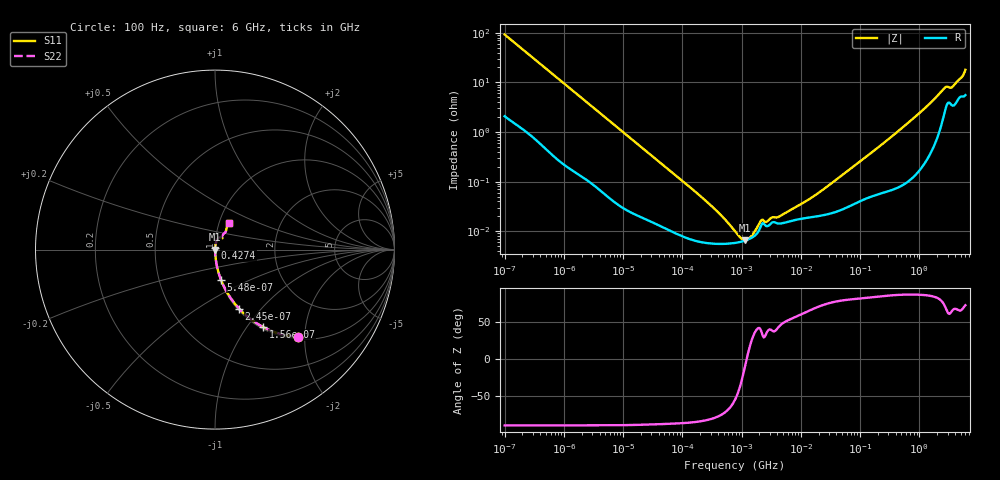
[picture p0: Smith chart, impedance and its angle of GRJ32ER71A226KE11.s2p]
!Murata Part Number: GRJ32ER71A226KE11
!These Parameters are Measured in Series Mode Connection
!Data Generated on Jun 19, 2026
!  o--ll--o
!Port1  Port2
!  o------o
!Operation Temp=25[degC], DC Bias Voltage=0[V]
!Freq. Start=100[Hz] Stop=6[GHz] 401[Steps]
# Hz S RI R 50
!Freq.(Hz) S11(Real) S11(Imag) S21(Real) S21(Imag) S12(Real) S12(Imag) S22(Real) S22(Imag)
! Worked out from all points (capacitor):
!   401 points, 100 Hz to 6 GHz, reference 50 ohm
!   read as one part in series: C = 17.1 uF near 109 Hz
!   lowest |Z| = 6.56 mohm at 1.159 MHz (marker M1)
!   series resonance near 1.218 MHz, so ESL is about 1 nH
!   S11 on the Smith chart (normalised r, x): 100 Hz: 1.04, -1.85; 156 Hz: 1.03, -1.19; 245 Hz: 1.02, -0.77; 548 Hz: 1.01, -0.35; 427.4 MHz: 1.00, +0.02; 6 GHz: 1.11, +0.34
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100  0.4622 -0.4874  0.5378 0.4874  0.5378 0.4874  0.4622 -0.4874
156  0.2664 -0.4304  0.7336 0.4304  0.7336 0.4304  0.2664 -0.4304
245  0.1342 -0.3286  0.8658 0.3286  0.8658 0.3286  0.1342 -0.3286
548  0.0329 -0.1671  0.9671 0.1671  0.9671 0.1671  0.0329 -0.1671
2008  0.00356 -0.0479  0.9964 0.0479  0.9964 0.0479  0.00356 -0.0479
40335  0.000137 -0.00252  0.9999 0.00252  0.9999 0.00252  0.000137 -0.00252
276587  5.73e-05 -0.000362  0.9999 0.000362  0.9999 0.000362  5.73e-05 -0.000362
774597  5.81e-05 -8.12e-05  0.9999 8.12e-05  0.9999 8.12e-05  5.81e-05 -8.12e-05
1159002  6.5e-05 -8.7e-06  0.9999 8.7e-06  0.9999 8.7e-06  6.5e-05 -8.7e-06
1585629  7.76e-05 4.75e-05  0.9999 -4.75e-05  0.9999 -4.75e-05  7.76e-05 4.75e-05
1734173  8.45e-05 6.53e-05  0.9999 -6.53e-05  0.9999 -6.53e-05  8.45e-05 6.53e-05
2169299  0.000135 0.0001  0.9999 -0.0001  0.9999 -0.0001  0.000135 0.0001
2713602  0.000126 9.44e-05  0.9999 -9.44e-05  0.9999 -9.44e-05  0.000126 9.44e-05
3245845  0.000149 0.000118  0.9999 -0.000118  0.9999 -0.000118  0.000149 0.000118
4440638  0.000143 0.000142  0.9999 -0.000142  0.9999 -0.000142  0.000143 0.000142
1.555665e7  0.000193 0.000444  0.9998 -0.000444  0.9998 -0.000444  0.000193 0.000444
3.124326e8  0.000704 0.00739  0.9993 -0.00739  0.9993 -0.00739  0.000704 0.00739
4.274388e8  0.000851 0.0101  0.9991 -0.0101  0.9991 -0.0101  0.000851 0.0101
1.251881e9  0.00332 0.0302  0.9967 -0.0302  0.9967 -0.0302  0.00332 0.0302
2.562649e9  0.0245 0.0678  0.9755 -0.0678  0.9755 -0.0678  0.0245 0.0678
3.666503e9  0.0379 0.0698  0.9621 -0.0698  0.9621 -0.0698  0.0379 0.0698
6e9  0.0768 0.1496  0.9232 -0.1496  0.9232 -0.1496  0.0768 0.1496
